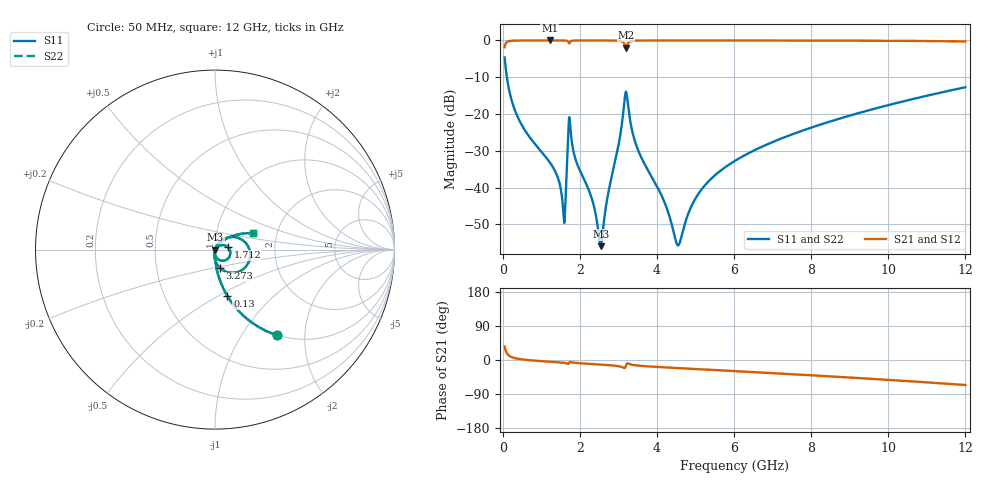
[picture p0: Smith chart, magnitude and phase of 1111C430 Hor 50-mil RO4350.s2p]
# GHz S MA R 50
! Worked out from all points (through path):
!   11951 points, 50 MHz to 12 GHz, reference 50 ohm
!   highest |S21| = -0.01 dB at 1.221 GHz (marker M1); lowest = -2.0 dB at 3.196 GHz (marker M2)
!   group delay of S21, straight-line fit = 15.8 ps
!   lowest |S11| = -55.9 dB at 2.541 GHz (marker M3), VSWR 1.00, Z = 50.2 - j0.0429 ohm
!   |S11| at or under -10 dB: 108.8 MHz to end of sweep
!   |S22| runs from -55.9 to -4.6 dB; largest |S21 - S12| = 0
!   S11 on the Smith chart (normalised r, x): 50 MHz: 0.99, -1.45; 130 MHz: 0.99, -0.56; 1.712 GHz: 1.16, +0.03; 3.273 GHz: 1.04, -0.22; 12 GHz: 1.51, +0.29
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0.05  0.5877 -54.2  0.8089 35.8  0.8089 35.8  0.5877 -54.2
0.13  0.2686 -75.0  0.9629 15.0  0.9629 15.0  0.2686 -75.0
0.455  0.07753 -87.4  0.9965 2.3  0.9965 2.3  0.07753 -87.4
1.221  0.02207 -92.5  0.9989 -4.6  0.9989 -4.6  0.02207 -92.5
1.44  0.01324 -91.1  0.9987 -6.1  0.9987 -6.1  0.01324 -91.1
1.583  0.003873 -53.3  0.9972 -7.4  0.9972 -7.4  0.003873 -53.3
1.629  0.006937 34.6  0.9948 -8.0  0.9948 -8.0  0.006937 34.6
1.712  0.07356 11.1  0.9308 -9.6  0.9308 -9.6  0.07356 11.1
1.759  0.06206 -67.8  0.9698 -5.2  0.9698 -5.2  0.06206 -67.8
2.042  0.01545 -92.8  0.9981 -8.8  0.9981 -8.8  0.01545 -92.8
2.325  0.006734 -88.7  0.9984 -10.7  0.9984 -10.7  0.006734 -88.7
2.541  0.001603 -15.5  0.9982 -12.1  0.9982 -12.1  0.001603 -15.5
3.196  0.2014 -15.7  0.7984 -15.0  0.7984 -15.0  0.2014 -15.7
3.273  0.1069 -74.5  0.9492 -9.9  0.9492 -9.9  0.1069 -74.5
3.495  0.03403 -95.4  0.9938 -14.6  0.9938 -14.6  0.03403 -95.4
4.034  0.009663 -96.8  0.9978 -18.5  0.9978 -18.5  0.009663 -96.8
4.555  0.001646 -16.7  0.9981 -21.4  0.9981 -21.4  0.001646 -16.7
5.086  0.008395 54.8  0.9981 -24.3  0.9981 -24.3  0.008395 54.8
6.025  0.02316 56.6  0.9977 -29.3  0.9977 -29.3  0.02316 56.6
8.017  0.06581 47.9  0.9954 -40.4  0.9954 -40.4  0.06581 47.9
10.009  0.1325 36.5  0.9882 -52.5  0.9882 -52.5  0.1325 36.5
12  0.2312 23.2  0.9692 -66.0  0.9692 -66.0  0.2312 23.2
